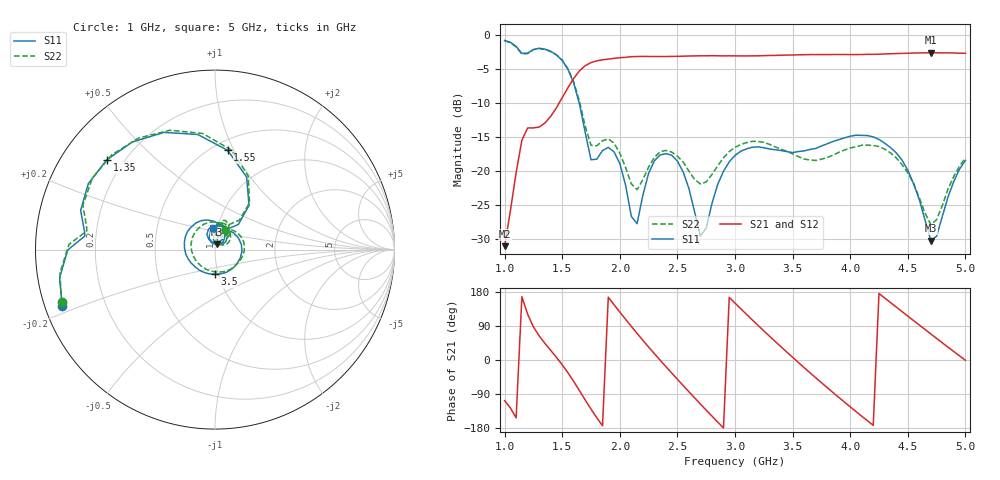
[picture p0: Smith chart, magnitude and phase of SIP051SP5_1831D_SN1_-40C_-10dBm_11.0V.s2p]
# GHz  S  dB  R  50
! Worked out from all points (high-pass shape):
!   81 points, 1 GHz to 5 GHz, reference 50 ohm
!   highest |S21| = -2.64 dB at 4.7 GHz (marker M1); lowest = -31.0 dB at 1 GHz (marker M2)
!   |S21| within 3 dB of the highest: 1.635 GHz to end of sweep
!   lowest |S11| = -30.2 dB at 4.7 GHz (marker M3), VSWR 1.06, Z = 51 + j2.97 ohm
!   |S11| at or under -10 dB: 1.647 GHz to end of sweep
!   |S22| runs from -27.8 to -0.9 dB; largest |S21 - S12| = 0.0017
!   S11 on the Smith chart (normalised r, x): 1 GHz: 0.05, -0.18; 1.35 GHz: 0.14, +0.36; 1.55 GHz: 0.59, +0.95; 3.5 GHz: 0.96, -0.27; 5 GHz: 0.95, +0.23
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1  -0.84 -159.7  -31.00 -107.2  -31.06 -107.8  -0.88 -161.0
1.15  -2.74 174.1  -15.46 166.9  -15.44 166.8  -2.83 171.7
1.35  -2.12 140.3  -12.94 43.9  -12.95 43.8  -2.15 137.4
1.55  -5.08 82.7  -7.75 -33.8  -7.75 -33.8  -5.00 80.7
1.7  -14.36 47.1  -4.54 -105.6  -4.54 -105.5  -13.42 50.4
1.85  -16.98 86.3  -3.68 -173.7  -3.67 -173.8  -15.54 76.7
2.05  -22.03 52.9  -3.31 107.5  -3.31 107.4  -19.46 51.6
2.15  -27.70 105.8  -3.20 70.1  -3.20 70.3  -22.72 75.4
2.35  -17.62 96.0  -3.20 -0.5  -3.19 -0.4  -17.16 77.7
2.5  -18.53 57.5  -3.17 -50.9  -3.16 -50.8  -17.79 52.0
2.65  -26.01 35.5  -3.11 -100.0  -3.10 -100.1  -21.24 45.9
2.7  -29.52 54.0  -3.09 -116.2  -3.08 -116.3  -21.87 53.3
2.85  -21.94 93.4  -3.09 -163.9  -3.10 -163.9  -19.21 64.5
3  -17.70 55.4  -3.10 150.1  -3.10 150.1  -16.52 45.1
3.25  -16.57 -18.4  -3.07 76.9  -3.06 76.9  -15.78 -3.7
3.5  -17.28 -91.1  -2.97 7.1  -2.97 7.1  -17.46 -65.1
3.7  -16.68 -139.7  -2.92 -46.6  -2.91 -46.6  -18.43 -128.9
3.95  -15.13 166.9  -2.90 -111.1  -2.89 -111.0  -16.91 152.2
4.15  -14.78 125.1  -2.88 -160.3  -2.88 -160.3  -16.18 100.4
4.35  -16.55 83.8  -2.79 151.6  -2.81 151.6  -17.32 57.5
4.7  -30.20 70.4  -2.64 68.7  -2.63 68.7  -27.85 47.3
5  -18.42 95.4  -2.73 -0.7  -2.73 -0.7  -18.07 62.2
